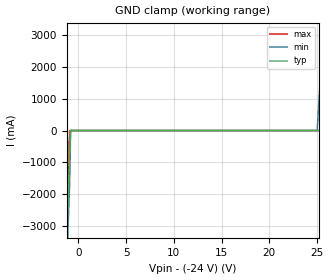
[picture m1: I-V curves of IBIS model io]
| TEXAS INSTRUMENTS INCORPORATED
| 1 Channel Uni-directional ESD-SURGE Protection Device
| Marketing Part #   Voltage Range   Package-type   #pins/pkg drawing
|   TSD24   -24V-24V   SOD-323   2/DYF
[IBIS Ver]   4.1
[Comment char]  |_char
[File Name]   tsd24.ibs
[File Rev]   1.0
"[Date]   Dec 20, 2023 "
[Source]   Data created from TI-SPICE simulations at TI-SLL/HVL.
   The following is an IBIS list for the TSD24.
   Please contact sllibis@ti.com with questions and
   comments concerning SLL IBIS models.
[Notes]
   - New measurements under nominal conditions only.
[Disclaimer]
"| TI and its licensors and suppliers make no warranties, either expressed"
"| or implied, with respect to this  model, including the warranties of "
"| provided solely on an ""as is"" basis. The entire risk as to its quality "
| and performance is with the customer.
[Copyright]
| (C) Copyright 2023 Texas Instruments Incorporated. All rights reserved.
| Component TSD24_DYF 2-PIN SOD-323
[Component]   TSD24_DYF
"[Manufacturer]   Texas Instruments, Inc."
[Package]   |2 SOD-323 - DYF package
   typ   min   max
R_pkg   20.0E-03   16.0E-03   24.0E-03
L_pkg   3.8E-10   3.0E-10   4.56E-10
C_pkg   5.7E-13   4.5E-13   6.8E-13
[Pin]   signal_name   model_name   R_pin   L_pin   C_pin
1   IO   io   2.07E-03   2.09E-10   6.95E-14
2   IO   io   2.07E-03   2.09E-10   6.95E-14
3   GND   gnd   2.07E-03   2.09E-10   6.95E-14
| Models and submodels in the file (1): io (Input)
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|   io Model
[Model]   io
Model_type  Input
| variable   typ   min   max
C_comp   16.5pF   13.2pF   19.8pF
[Voltage Range]   24   20   28
[Temperature Range]   27   -55   150
[Power Clamp Reference]   0   0   0
[GND Clamp Reference]   -24   -20   -28
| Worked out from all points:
|   GND clamp passes 1 mA (typ) near -0.80 V on its own axis
[GND Clamp]
|	Voltage	  I(typ)	  I(min)   I(max)
-3V       -18.3A     -19.2A     -17.5A
-1.3V     -4.17A     -5A        -3.33A
-1.1V     -2.5A      -3.33A     -1.67A
-900mV    -833mA     -1.67A     13.9fA
-800mV    -5nA       -5nA       -5nA
25V       4.1nA      4.1nA      4.1nA
26V       4.26nA     5A         4.26nA
30V       4.92nA     45A        4.92nA
31V       5A         55A        5.08nA
35V       45A        95A        5.74nA
36V       55A        105A       5A
50V       195A       245A       145A
[Power Clamp]
|   Voltage   I(typ)   I(min)   I(max)
-24V      0A         0A         0A
0V        0A         0A         0A
24V       0A         0A         0A
